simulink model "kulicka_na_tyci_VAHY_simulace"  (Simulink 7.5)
settings: Solver=ode45  StartTime=0.0  StopTime=100  RelTol=1e-3
undefined symbols (not defined in the file or in its folder): KA, KB, KC, KD
libraries: mathlib x25, execlib x1

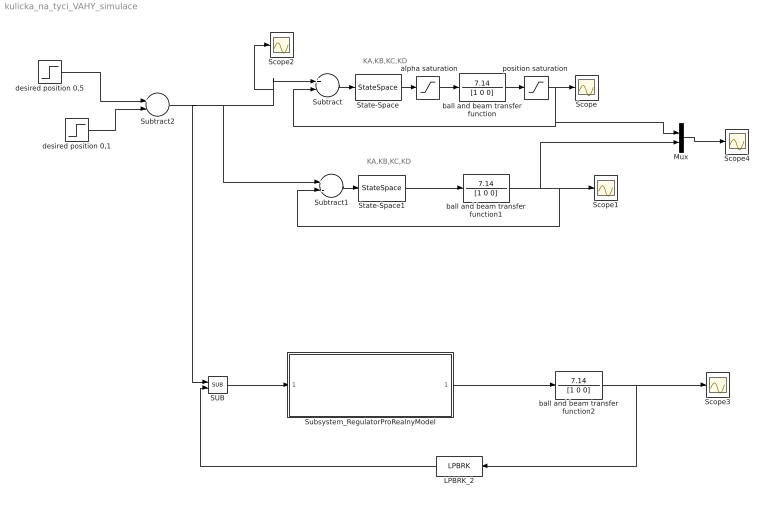
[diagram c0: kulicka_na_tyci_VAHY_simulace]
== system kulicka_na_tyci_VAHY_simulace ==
  note: KA,KB,KC,KD
  note: KA,KB,KC,KD
  " alpha saturation" : Saturate  UpperLimit=0.01  LowerLimit=-0.01
  LPBRK_2 : execlib/LPBRK
  Mux : Mux  Inputs=2
  SUB : mathlib/SUB  SystemSampleTime=-1
  Scope{,1..4} (5 alike) : Scope
  State-Space : StateSpace  A=KA  B=KB  C=KC  D=KD
  State-Space1 : StateSpace  A=KA  B=KB  C=KC  D=KD
  Subsystem_RegulatorProRealnyModel : Subsystem
  Subtract : Sum  Inputs=+-  OutDataType=sfix(16)  OutScaling=2^-10
  Subtract1 : Sum  Inputs=+-  OutDataType=sfix(16)  OutScaling=2^-10
  Subtract2 : Sum  Inputs=+-  OutDataType=sfix(16)  OutScaling=2^-10
  ball and beam transfer function : TransferFcn  Numerator=7.14  Denominator=[1 0 0]
  ball and beam transfer function1 : TransferFcn  Numerator=7.14  Denominator=[1 0 0]
  ball and beam transfer function2 : TransferFcn  Numerator=7.14  Denominator=[1 0 0]
  desired position 0,1 : Step  Time=50  After=0.4  SampleTime=0
  desired position 0,5 : Step  Time=0  After=0.5  SampleTime=0
  "position saturation " : Saturate  UpperLimit=0.95  LowerLimit=0
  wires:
  State-Space/1 -> " alpha saturation"/1
  ball and beam transfer function/1 -> "position saturation "/1
  Subtract/1 -> State-Space/1
  " alpha saturation"/1 -> ball and beam transfer function/1
  "position saturation "/1 -> Scope/1, Subtract/2, Mux/1
  State-Space1/1 -> ball and beam transfer function1/1
  ball and beam transfer function1/1 -> Subtract1/2, Scope1/1, Mux/2
  Subtract1/1 -> State-Space1/1
  desired position 0,5/1 -> Subtract2/1
  Subtract2/1 -> SUB/1, Subtract/1, Scope2/1, Subtract1/1
  desired position 0,1/1 -> Subtract2/2
  ball and beam transfer function2/1 -> Scope3/1, LPBRK_2/1
  SUB/1 -> Subsystem_RegulatorProRealnyModel/1(e)
  Subsystem_RegulatorProRealnyModel/1(u) -> ball and beam transfer function2/1
  LPBRK_2/1 -> SUB/2
  Mux/1 -> Scope4/1

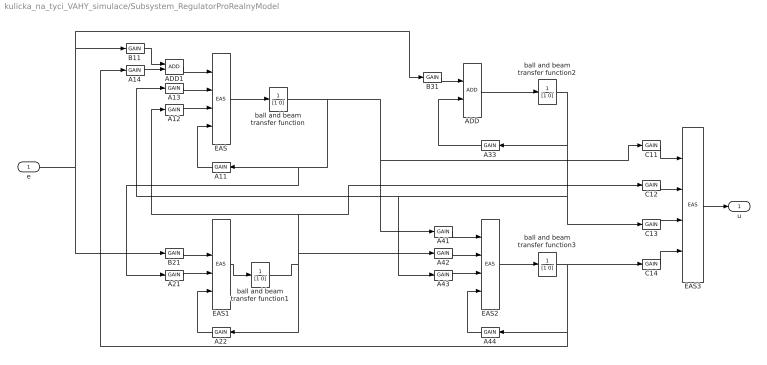
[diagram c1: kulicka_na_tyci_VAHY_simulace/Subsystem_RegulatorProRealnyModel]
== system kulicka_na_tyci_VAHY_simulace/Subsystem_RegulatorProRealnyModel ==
  e : Inport
  A11 : mathlib/GAIN  SystemSampleTime=-1  k=-0.3206
  A12 : mathlib/GAIN  SystemSampleTime=-1  k=-818.6
  A13 : mathlib/GAIN  SystemSampleTime=-1  k=-0.1872
  A14 : mathlib/GAIN  SystemSampleTime=-1  k=14.99
  A21 : mathlib/GAIN  SystemSampleTime=-1  k=0.0009766
  A22 : mathlib/GAIN  SystemSampleTime=-1  k=-1.194
  A33 : mathlib/GAIN  SystemSampleTime=-1  k=-0.00025
  A41 : mathlib/GAIN  SystemSampleTime=-1  k=-20.45
  A42 : mathlib/GAIN  SystemSampleTime=-1  k=-5679
  A43 : mathlib/GAIN  SystemSampleTime=-1  k=-11.98
  A44 : mathlib/GAIN  SystemSampleTime=-1  k=-40.8
  ADD : mathlib/ADD  SystemSampleTime=-1
  ADD1 : mathlib/ADD  SystemSampleTime=-1
  B11 : mathlib/GAIN  SystemSampleTime=-1  k=-1067
  B21 : mathlib/GAIN  SystemSampleTime=-1  k=-1.745
  B31 : mathlib/GAIN  SystemSampleTime=-1  k=-83.5
  C11 : mathlib/GAIN  SystemSampleTime=-1  k=-0.0000299
  C12 : mathlib/GAIN  SystemSampleTime=-1  k=-0.008302
  C13 : mathlib/GAIN  SystemSampleTime=-1  k=-0.00001751
  C14 : mathlib/GAIN  SystemSampleTime=-1  k=0.001402
  EAS{,1..3} (4 alike) : mathlib/EAS  SystemSampleTime=-1  a=1  b=1  c=1  d=1  y0=0
  ball and beam transfer function{,1..3} (4 alike) : TransferFcn  Numerator=1  Denominator=[1 0]
  u : Outport
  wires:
  A11/1 -> EAS/4
  A12/1 -> EAS/3
  A13/1 -> EAS/2
  A14/1 -> ADD1/2
  A21/1 -> EAS1/3
  A22/1 -> EAS1/4
  A33/1 -> ADD/2
  A41/1 -> EAS2/1
  A42/1 -> EAS2/2
  A43/1 -> EAS2/3
  A44/1 -> EAS2/4
  ADD/1 -> ball and beam transfer function2/1
  ADD1/1 -> EAS/1
  B11/1 -> ADD1/1
  B21/1 -> EAS1/2
  B31/1 -> ADD/1
  C11/1 -> EAS3/1
  C12/1 -> EAS3/2
  C13/1 -> EAS3/3
  C14/1 -> EAS3/4
  EAS3/1 -> u/1
  e/1 -> B21/1, B11/1, B31/1
  EAS/1 -> ball and beam transfer function/1
  EAS2/1 -> ball and beam transfer function3/1
  ball and beam transfer function3/1 -> C14/1, A44/1, A14/1
  ball and beam transfer function1/1 -> A22/1, A42/1, A12/1, C12/1
  ball and beam transfer function2/1 -> A33/1, C13/1, A13/1, A43/1
  ball and beam transfer function/1 -> A41/1, C11/1, A21/1, A11/1
  EAS1/1 -> ball and beam transfer function1/1
